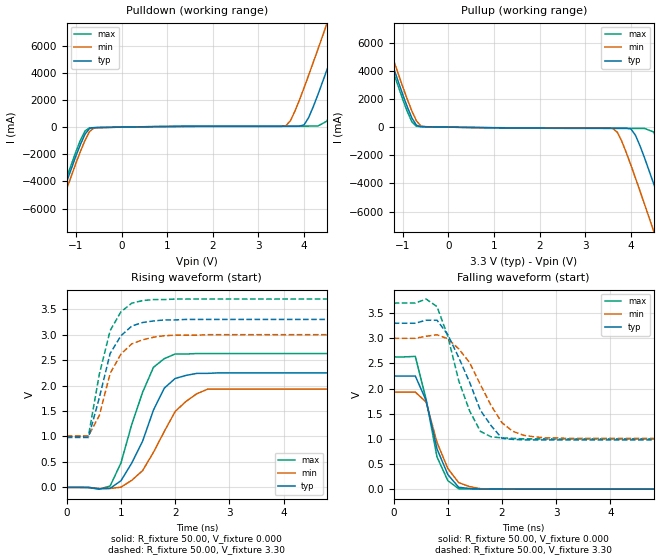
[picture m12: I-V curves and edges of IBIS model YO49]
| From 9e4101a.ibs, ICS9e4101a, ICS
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|   Model YO49
[Model]   YO49
Model_type   Output
Polarity   Non-Inverting
C_comp   5.50pF   5.00pF   6.00pF
[Temperature Range]   27.00   70.00   0.000
[Voltage Range]   3.30V   3.00V   3.70V
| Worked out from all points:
|   slope of the pulldown table from 0 to 0.495 V, typ, clamps not added: 18 ohm
|   slope of the pullup table from 0 to 0.495 V, typ, clamps not added: 20.5 ohm
|   rising waveform, R_fixture 50.00, V_fixture 0.000: 20-80 % time 547ps typ, 623ps min, 483ps max; typ from 0 V to 2.25 V
|   rising waveform, R_fixture 50.00, V_fixture 3.30: 20-80 % time 399ps typ, 392ps min, 356ps max; typ from 0.98 V to 3.3 V
|   falling waveform, R_fixture 50.00, V_fixture 0.000: 20-80 % time 354ps typ, 371ps min, 324ps max; typ from 2.25 V to 0 V
|   falling waveform, R_fixture 50.00, V_fixture 3.30: 20-80 % time 577ps typ, 609ps min, 450ps max; typ from 3.3 V to 0.98 V
[Pulldown]
| voltage   I(typ)   I(min)   I(max)
-3.3V     -24.49A    -24.99A    -24.19A
-1.7V     -8.76A     -9.29A     -8.44A
-1.5V     -6.83A     -7.35A     -6.5A
-900mV    -1.27A     -1.78A     -960mA
-700mV    -92.15mA   -320mA     -52.86mA
3.6V      62.06mA    99.79mA    76.5mA
4V        170mA      2.9A       76.74mA
4.3V      2.36A      5.7A       77.36mA
4.5V      4.21A      7.62A      440mA
4.9V      8.05A      11.49A     3.88A
5.3V      11.94A     15.41A     7.72A
6.6V      24.78A     28.25A     20.51A
[Pullup]
| voltage   I(typ)   I(min)   I(max)
-3.3V     24.69A     25.21A     24.36A
-1.7V     8.95A      9.5A       8.61A
-1.5V     7.02A      7.57A      6.67A
-900mV    1.43A      1.97A      1.1A
-700mV    130mA      440mA      60.77mA
-500mV    27.78mA    26.61mA    30.44mA
3.6V      -71.61mA   -83.61mA   -90.07mA
4V        -130mA     -2.71A     -91.27mA
4.5V      -4.04A     -7.41A     -350mA
4.9V      -7.87A     -11.28A    -3.73A
5.3V      -11.76A    -15.2A     -7.56A
6.6V      -24.57A    -28.02A    -20.33A
[Ramp]
| variable   typ   min   max
dV/dt_r   1.35/0.48n   1.16/0.59n   1.58/0.40n
dV/dt_f   1.39/0.52n   1.19/0.58n   1.62/0.38n
R_load = 50.00
[Rising Waveform]
R_fixture = 50.00
V_fixture = 0.000
V_fixture_min = 0.000
V_fixture_max = 0.000
| time   V(typ)   V(min)   V(max)
0s        0V         0V         0V
800ps     -18.14mV   -21.27mV   27.31mV
1ns       130mV      3.99mV     480mV
1.2ns     480mV      140mV      1.24V
1.4ns     910mV      330mV      1.87V
1.6ns     1.52V      690mV      2.36V
1.8ns     1.95V      1.1V       2.53V
2ns       2.14V      1.49V      2.62V
2.6ns     2.24V      1.93V      2.63V
10ns      2.25V      1.93V      2.63V
[Rising Waveform]
R_fixture = 50.00
V_fixture = 3.30
V_fixture_min = 3.00
V_fixture_max = 3.70
| time   V(typ)   V(min)   V(max)
0s        980mV      1.01V      1V
400ps     980mV      1.01V      1.01V
600ps     1.76V      1.41V      2.22V
800ps     2.63V      2.24V      3.08V
1ns       2.98V      2.62V      3.45V
1.2ns     3.17V      2.82V      3.62V
1.4ns     3.24V      2.9V       3.67V
1.6ns     3.27V      2.95V      3.69V
2ns       3.29V      2.99V      3.7V
10ns      3.3V       3V         3.7V
[Falling Waveform]
R_fixture = 50.00
V_fixture = 0.000
V_fixture_min = 0.000
V_fixture_max = 0.000
| time   V(typ)   V(min)   V(max)
0s        2.25V      1.93V      2.63V
400ps     2.25V      1.93V      2.64V
600ps     1.76V      1.73V      1.78V
800ps     800mV      930mV      640mV
1ns       290mV      410mV      170mV
1.2ns     37.2mV     130mV      7.42mV
1.4ns     13.61mV    51.13mV    4.51mV
1.6ns     1.96mV     9.67mV     2.07mV
1.8ns     1.77mV     3.5mV      1.06mV
10ns      0V         0V         -4.02uV
[Falling Waveform]
R_fixture = 50.00
V_fixture = 3.30
V_fixture_min = 3.00
V_fixture_max = 3.70
| time   V(typ)   V(min)   V(max)
0s        3.3V       3V         3.7V
600ps     3.36V      3.04V      3.78V
800ps     3.36V      3.07V      3.63V
1ns       3.07V      2.99V      3.04V
1.4ns     2.13V      2.52V      1.56V
1.6ns     1.57V      2.08V      1.15V
1.8ns     1.26V      1.66V      1.04V
2.2ns     990mV      1.15V      1.01V
2.8ns     980mV      1.02V      1V
10ns      980mV      1.01V      1V
